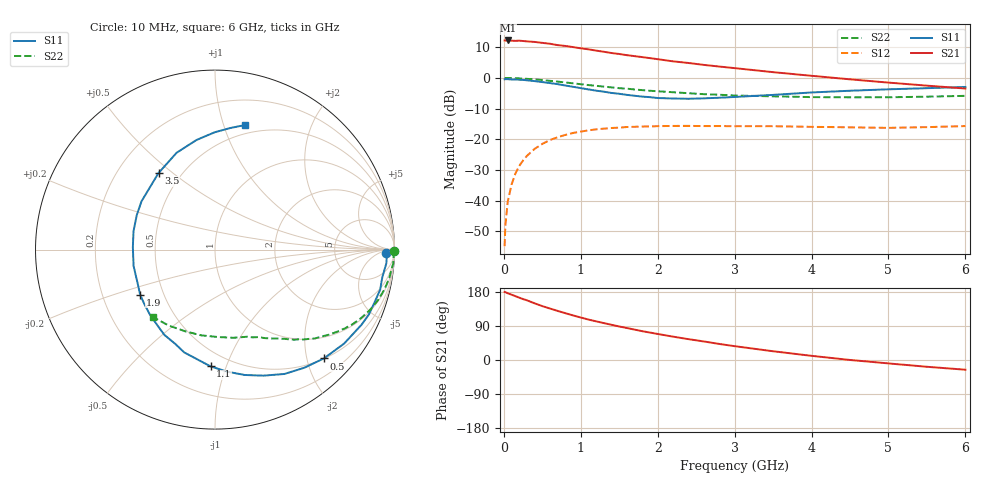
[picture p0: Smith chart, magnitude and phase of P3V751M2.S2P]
! SIEMENS Small Signal Semiconductors
! BFP181
! Si NPN RF Bipolar Junction Transistor in SOT143
! VCE = 0.75 V  IC = 1.2 mA
! Common Emitter S-Parameters:  March  1996
# GHz  S  MA  R  50
!  f  S11  S21  S12  S22
! GHz  MAG  ANG  MAG  ANG  MAG  ANG  MAG  ANG
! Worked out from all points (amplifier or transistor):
!   36 points, 10 MHz to 6 GHz, reference 50 ohm
!   highest |S21| = 12.3 dB at 50 MHz (marker M1)
!   |S21| within 3 dB of that: start of sweep to 1.125 GHz
!   unconditionally stable (mu >= 1): 2.643 GHz to end of sweep
!   at 250 MHz: K = 0.10, MSG = 19.5 dB, |S12| = -26.9 dB
!   at 1.4 GHz: K = 0.58, MSG = 12.2 dB, |S12| = -16.3 dB
!   at 6 GHz: K = 1.37, MAG = 2.5 dB, |S12| = -15.7 dB
!   S11 on the Smith chart (normalised r, x): 10 MHz: 35, -13; 500 MHz: 0.51, -2.32; 1.1 GHz: 0.39, -0.88; 1.9 GHz: 0.37, -0.24; 3.5 GHz: 0.38, +0.45; 6 GHz: 0.42, +1.18
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0.01  0.9506 -1.1  4.096 179.5  0.0018 84.6  0.9978 -0.4
0.02  0.9579 -2.3  4.079 179.1  0.0039 88.0  0.9959 -0.9
0.05  0.9576 -4.6  4.098 176.2  0.0095 90.5  0.9959 -2.3
0.1  0.9448 -9.4  4.064 172.4  0.0182 83.1  0.9962 -4.5
0.2  0.9361 -18.4  4.065 164.5  0.0367 77.8  0.9846 -9.0
0.4  0.8896 -36.1  3.878 149.5  0.0697 66.8  0.9495 -17.5
0.5  0.8576 -45.0  3.743 142.2  0.084 61.5  0.9257 -21.4
0.6  0.8252 -52.9  3.621 135.8  0.0972 56.4  0.8991 -25.1
0.8  0.7527 -68.9  3.335 123.5  0.1177 47.4  0.8457 -31.3
0.9  0.7178 -76.7  3.196 117.6  0.1267 43.3  0.8183 -34.1
1.1  0.6511 -92.2  2.936 106.7  0.1397 36.0  0.7663 -39.2
1.3  0.5981 -106.6  2.678 97.4  0.149 29.8  0.7225 -43.5
1.5  0.5526 -120.7  2.465 88.4  0.1547 24.8  0.6822 -47.1
1.9  0.4866 -149.0  2.109 72.4  0.162 16.6  0.6184 -53.4
2.2  0.4627 -168.7  1.87 61.6  0.1652 11.9  0.5852 -57.8
2.4  0.4579 178.2  1.758 55.0  0.1654 8.9  0.5647 -60.8
2.8  0.4762 156.3  1.538 42.4  0.1643 5.0  0.5329 -66.6
3.5  0.5301 126.4  1.245 23.1  0.1633 -0.5  0.5022 -78.0
4  0.5805 111.6  1.086 11.0  0.1596 -3.1  0.4874 -88.0
4.5  0.6193 99.6  0.951 0.1  0.1565 -5.1  0.4838 -99.0
5.5  0.682 83.0  0.75 -17.9  0.1578 -4.0  0.4955 -121.4
6  0.7141 76.4  0.673 -25.6  0.1642 -4.1  0.5113 -132.8
